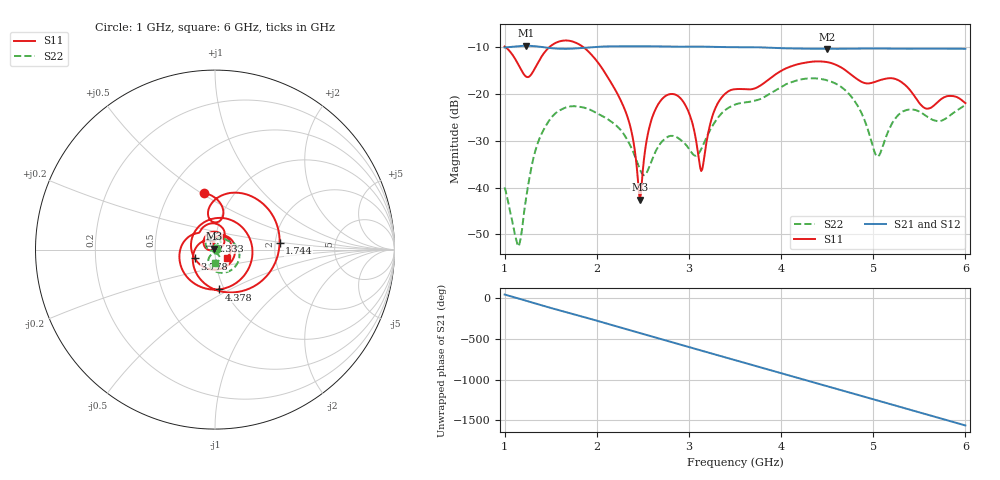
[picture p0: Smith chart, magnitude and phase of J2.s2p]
!Agilent Technologies,E8364B,MY43040528,A.07.50.67
!Agilent E8364B: A.07.50.67
!Date: Sunday, March 01, 2026 15:21:52
!Correction: S11(Full 2 Port(1,2))
!S21(Full 2 Port(1,2))
!S12(Full 2 Port(1,2))
!S22(Full 2 Port(1,2))
!S2P File: Measurements: S11, S21, S12, S22:
# Hz S  dB  R 50
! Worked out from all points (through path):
!   451 points, 1 GHz to 6 GHz, reference 50 ohm
!   highest |S21| = -9.69 dB at 1.233 GHz (marker M1); lowest = -10.4 dB at 4.5 GHz (marker M2)
!   group delay of S21, straight-line fit = 893 ps
!   lowest |S11| = -42.6 dB at 2.467 GHz (marker M3), VSWR 1.01, Z = 49.5 + j0.533 ohm
!   |S11| at or under -10 dB: 1.011 GHz to 1.485 GHz (474.4 MHz wide, 38 % of centre); 1.856 GHz to end of sweep
!   |S22| runs from -52.5 to -16.7 dB; largest |S21 - S12| = 0.0016
!   S11 on the Smith chart (normalised r, x): 1 GHz: 0.73, +0.51; 1.744 GHz: 2.11, +0.18; 2.333 GHz: 0.94, +0.10; 3.778 GHz: 0.79, -0.08; 4.378 GHz: 0.94, -0.44; 6 GHz: 1.14, -0.10
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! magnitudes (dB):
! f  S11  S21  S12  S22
! 1 GHz  -9.8  -10.1  -10.1  -40.0
! 1.144 GHz  -13.5  -9.8  -9.8  -52.5
! 1.233 GHz  -16.3  -9.7  -9.7  -42.2
! 1.411 GHz  -11.7  -10.0  -10.0  -28.1
! 1.744 GHz  -8.8  -10.3  -10.3  -22.6
! 1.844 GHz  -9.8  -10.2  -10.2  -22.8
! 2.333 GHz  -24.9  -9.8  -9.8  -29.9
! 2.467 GHz  -42.6  -9.8  -9.8  -36.1
! 2.667 GHz  -22.2  -9.8  -9.9  -31.3
! 2.933 GHz  -21.5  -9.9  -9.9  -30.2
! 3.133 GHz  -36.5  -9.9  -9.9  -31.8
! 3.289 GHz  -22.9  -9.9  -10.0  -25.8
! 3.5 GHz  -19.0  -10.0  -10.0  -22.3
! 3.778 GHz  -18.2  -10.0  -10.1  -21.1
! 4.344 GHz  -13.1  -10.3  -10.4  -16.7
! 4.378 GHz  -13.0  -10.3  -10.4  -16.7
! 4.5 GHz  -13.2  -10.4  -10.4  -17.1
! 4.811 GHz  -16.6  -10.3  -10.3  -21.9
! 5.033 GHz  -17.3  -10.3  -10.3  -33.2
! 5.167 GHz  -16.6  -10.3  -10.4  -27.8
! 5.567 GHz  -23.1  -10.3  -10.3  -24.6
! 6 GHz  -22.0  -10.3  -10.4  -22.3
